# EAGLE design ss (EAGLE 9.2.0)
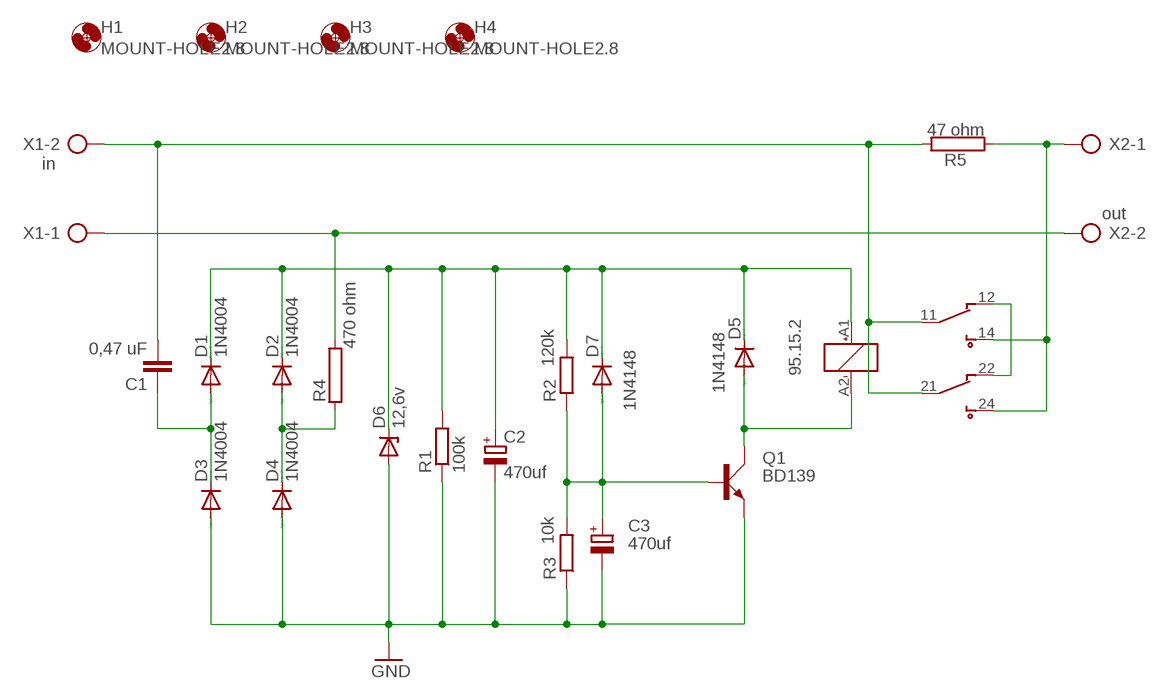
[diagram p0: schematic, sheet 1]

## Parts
C1  0,47 uF  C-EU225-108X268  [C225-108X268]
C2  470uf  CPOL-EUE2.5-7  [E2,5-7]
C3  470uf  CPOL-EUE3.5-8  [E3,5-8]
D1  1N4004  [DO41-10]
D2  1N4004  [DO41-10]
D3  1N4004  [DO41-10]
D4  1N4004  [DO41-10]
D5  1N4148  1N4148DO35-7  [DO35-7]
D6  12,6v  ZENER-DIODEDO34-7  [DO34Z7]
D7  1N4148  1N4148DO35-7  [DO35-7]
H1  MOUNT-HOLE2.8  [2,8]
H2  MOUNT-HOLE2.8  [2,8]
H3  MOUNT-HOLE2.8  [2,8]
H4  MOUNT-HOLE2.8  [2,8]
Q1  BD139  [TO126AV]
R1  100k  R-EU_0207/10  [0207/10]
R2  120k  R-EU_0207/10  [0207/10]
R3  10k  R-EU_0207/10  [0207/10]
R4  470 ohm  RAC01  [AC01]
R5  47 ohm  RHS10  [HS10]
RL1  95.15.2  [95.15.2]
X1  in  AK300/2  [AK300/2]
X2  out  AK300/2  [AK300/2]

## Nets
GND: C2.- C3.- D3.A D4.A D6.A Q1.E R1.1 R3.1
N$1: RL1.12 RL1.22
N$2: R5.1 RL1.14 RL1.24 X2.1
N$3: R4.2 X1.1 X2.2
N$4: C1.1 D1.A D3.C
N$5: D2.A D4.C R4.1
N$6: C2.+ D1.C D2.C D5.C D6.C D7.C R1.2 R2.2 RL1.A1
N$8: C3.+ D7.A Q1.B R2.1 R3.2
N$10: D5.A Q1.C RL1.A2
N$12: C1.2 R5.2 RL1.11 RL1.21 X1.2

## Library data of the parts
C1 = rcl:C-EU: CAPACITOR, European symbol
C2 C3 = rcl:CPOL-EU: POLARIZED CAPACITOR, European symbol
D1-D4 = diode:1N4004: DIODE
D5 D7 = diode:1N4148: DIODE
D6 = diode:ZENER-DIODE: Z-Diode
H1-H4 = holes:MOUNT-HOLE: MOUNTING HOLE with drill center marker
Q1 = transistor-power:BD139: NPN TRANSISTOR
R1-R3 = rcl:R-EU_: RESISTOR, European symbol
R4 = resistor-power:R: Power Resitor; OC_FARNELL: unknown; OC_NEWARK: unknown
R5 = resistor-power:R: Power Resitor; MF: OHMITE; MPN: RHS10K; OC_FARNELL: 1050333; OC_NEWARK: 01F7568
RL1 = relay_finder_36_11:95.15.2: P.C.B. socket suitable for the 40.51 & 40.52 & 40.61 relays
X1 X2 = con-ptr500:AK300/2: CONNECTOR; OC_FARNELL: unknown; OC_NEWARK: unknown

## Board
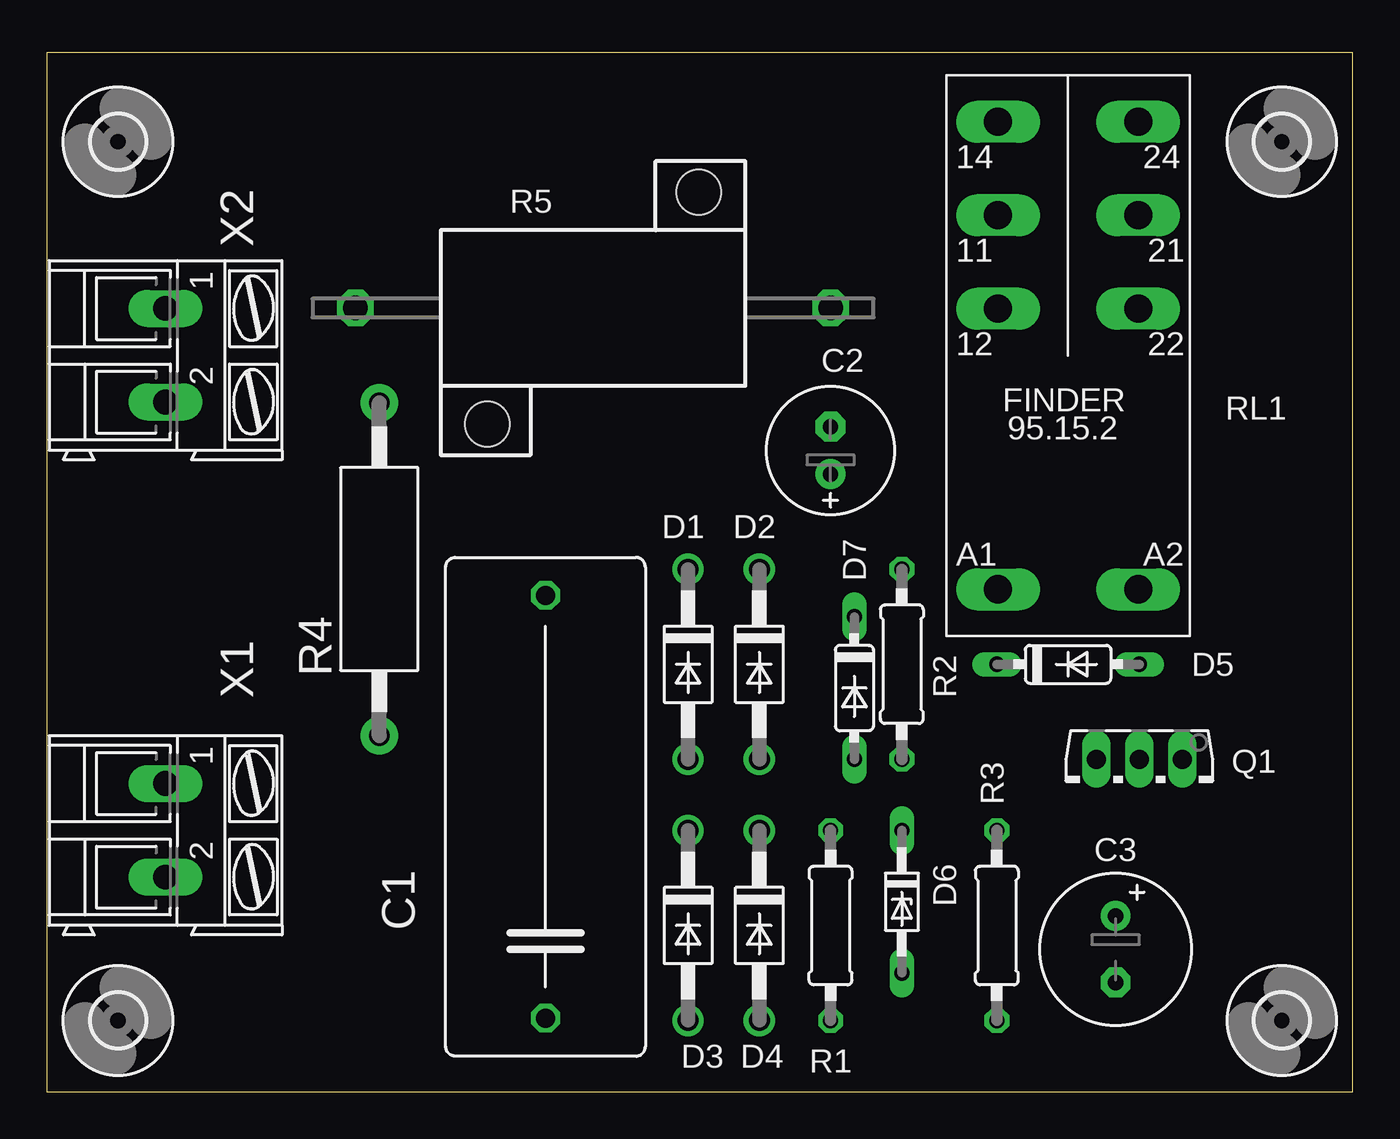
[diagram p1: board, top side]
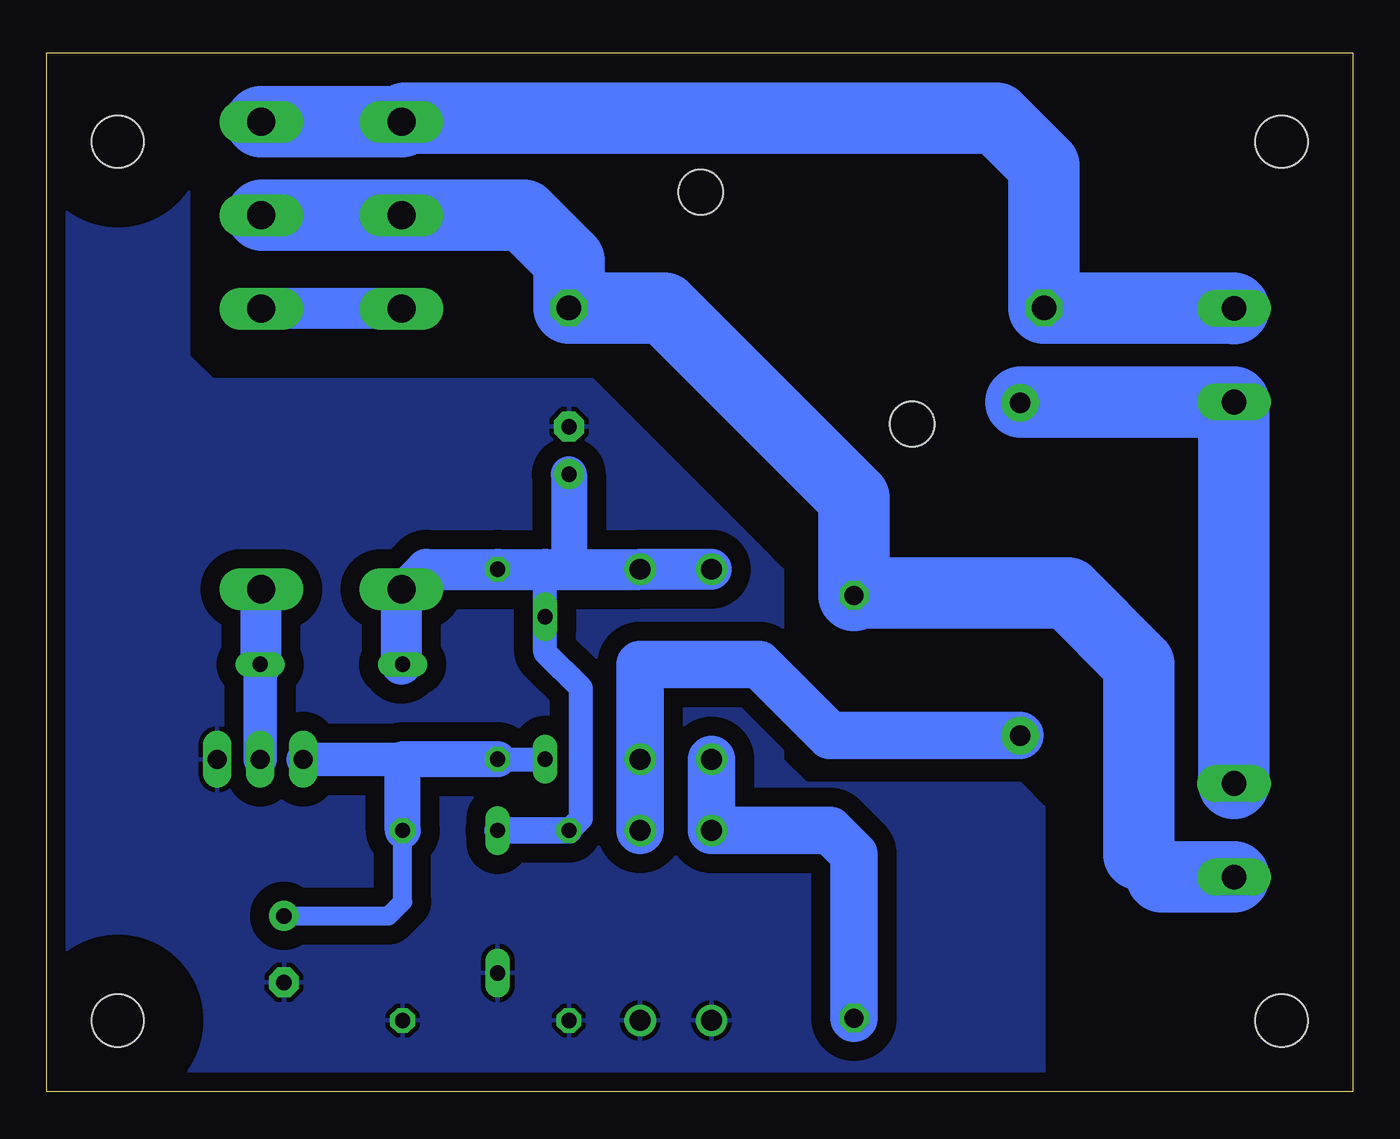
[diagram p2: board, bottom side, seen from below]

Size 69.83 x 55.55 mm. Coordinates in mm from the lower left corner, seen from the top.
Outline: 0,0 69.83,0 69.83,55.55 0,55.55 0,0
Copper layers (1*16): Top 0.035mm / dielectric 1.5mm / Bottom 0.035mm
Design rules "default": minimum track width 10mil, minimum drill 24mil, track to track 8mil, track to pad 8mil, pad to pad 8mil, via to via 8mil, smd to smd 8mil, copper to edge 40mil, drill to drill 8mil, minimum pad ring 10mil, minimum via ring 8mil, stop-mask expansion 4mil, vias tented up to drill 0mil, thermal gap 10mil

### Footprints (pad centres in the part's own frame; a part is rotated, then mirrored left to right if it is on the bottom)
C225-108X268 = drill 1.016 octagon: 1 -11.303,0; 2 11.303,0
E2,5-7 = drill 0.813 pad 1.6: + -1.27,0 | drill 0.813 pad 1.6 octagon: - 1.27,0
E3,5-8 = drill 0.813 pad 1.6: + -1.778,0 | drill 0.813 pad 1.6 octagon: - 1.778,0
DO41-10 = drill 1.118: A 5.08,0; C -5.08,0
DO35-7 = drill 0.813 long: A 3.81,0; C -3.81,0
DO34Z7 = drill 0.813 long: A 3.81,0; C -3.81,0
2,8 = hole 2.8: 0,0
TO126AV = drill 1.016 long: B 2.286,-1.27; C 0,-1.27; E -2.286,-1.27
0207/10 = drill 0.813 octagon: 1 -5.08,0; 2 5.08,0
AC01 = drill 1.1 pad 2: 1 -8.9,0; 2 8.9,0
HS10 = drill 1.3 octagon: 1 -12.7,0; 2 12.7,0 | hole 2.4: -5.65,-6.2; 5.65,6.2
95.15.2 = drill 1.5 long: 11 -3.75,7.5; 12 -3.75,2.5; 14 -3.75,12.5; 21 3.75,7.5; 22 3.75,2.5; 24 3.75,12.5; A1 -3.75,-12.5; A2 3.75,-12.5
AK300/2 = drill 1.321 long: 1 -2.515,0; 2 2.489,0

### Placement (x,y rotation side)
C1  26.67,15.24 90 top
C2  41.91,34.29 90 top
C3  57.15,7.62 270 top
D1  34.29,22.86 270 top
D2  38.1,22.86 270 top
D3  34.29,8.89 270 top
D4  38.1,8.89 270 top
D5  54.61,22.86 0 top
D6  45.72,10.16 270 top
D7  43.18,21.59 270 top
H1  66.04,50.8 0 top
H2  66.04,3.81 0 top
H3  3.81,3.81 0 top
H4  3.81,50.8 0 top
Q1  58.42,16.51 180 top
R1  41.91,8.89 90 top
R2  45.72,22.86 90 top
R3  50.8,8.89 90 top
R4  17.78,27.94 90 top
R5  29.21,41.91 0 top
RL1  54.61,39.37 0 top
X1  6.35,13.97 270 top
X2  6.35,39.37 270 top

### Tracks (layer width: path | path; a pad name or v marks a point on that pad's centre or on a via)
GND
  Bottom 1.016: 60.96,17.53 Q1.E
  pour Bottom (isolate 1.016): 16.51,0 68.58,0 69.85,1.27 69.85,53.34 68.58,54.61 63.5,54.61 62.23,53.34 62.23,39.37 60.96,38.1 40.64,38.1 39.37,36.83 31.75,29.21 30.48,27.94 30.48,17.78 29.21,16.51 24.13,16.51 17.78,16.51 16.51,15.24
N$1
  Bottom 2.184: RL1.12 RL1.22
N$2
  Bottom 1.422: 50.66,52.07 RL1.14
  Bottom 3.81: X2.1 6.38,41.91 R5.1 16.51,49.53 19.05,52.07 50.66,52.07 | RL1.14 RL1.24
N$3
  Bottom 1.016: 6.39,35.57 X2.2
  Bottom 2.184: 17.74,36.88 R4.2
  Bottom 3.81: X1.1 X2.2 17.74,36.88
N$4
  Bottom 2.54: C1.1 26.67,12.7 27.94,13.97 D3.C D1.A
N$5
  Bottom 1.422: R4.1
  Bottom 2.54: D4.C D2.A 38.1,22.86 31.75,22.86 27.94,19.05 R4.1
N$6
  Bottom 1.27: 43.18,27.94 D7.C 43.18,23.5 41.27,21.59 41.27,14.61 R1.2
  Bottom 1.422: D6.C R1.2 | D5.C 50.86,22.86
  Bottom 1.93: C2.+ 41.91,27.94
  Bottom 2.184: D1.C D2.C 41.91,27.94 43.18,27.94 R2.2 49.53,27.94 50.6,26.87 RL1.A1 50.86,22.86
N$8
  Bottom 1.016: C3.+ 51.56,9.4 50.8,10.16 R3.2
  Bottom 1.27: R2.1 D7.A
  Bottom 1.778: 50.8,17.78 Q1.B
  Bottom 1.93: R2.1 50.8,17.78 R3.2
N$10
  Bottom 1.422: D5.A 58.36,22.86
  Bottom 1.778: Q1.C D5.A
  Bottom 2.184: 58.36,22.86 RL1.A2
N$12
  Bottom 1.016: 10.21,11.48 11.43,12.7 | 26.54,26.67 C1.2 | 58.3,46.87 58.42,46.99 58.42,46.93 RL1.21
  Bottom 3.81: X1.2 10.21,11.48 | 11.43,12.7 11.43,22.86 15.24,26.67 26.54,26.67 | 58.3,46.87 RL1.11 44.33,46.87 41.91,44.45 R5.2 36.83,41.91 26.67,31.75 C1.2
